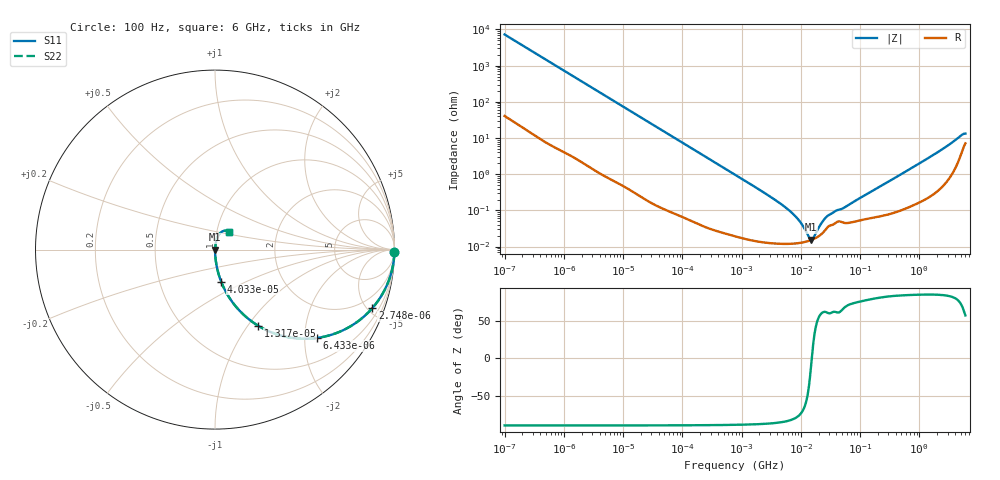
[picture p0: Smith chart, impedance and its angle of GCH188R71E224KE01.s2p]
!Murata Part Number: GCH188R71E224KE01
!These Parameters are Measured in Series Mode Connection
!Data Generated on Jun 19, 2026
!  o--ll--o
!Port1  Port2
!  o------o
!Operation Temp=25[degC], DC Bias Voltage=0[V]
!Freq. Start=100[Hz] Stop=6[GHz] 401[Steps]
# Hz S RI R 50
!Freq.(Hz) S11(Real) S11(Imag) S21(Real) S21(Imag) S12(Real) S12(Imag) S22(Real) S22(Imag)
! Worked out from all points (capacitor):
!   401 points, 100 Hz to 6 GHz, reference 50 ohm
!   read as one part in series: C = 218 nF near 109 Hz
!   lowest |Z| = 15.4 mohm at 14.88 MHz (marker M1)
!   series resonance near 15.31 MHz, so ESL is about 490 pH
!   S11 on the Smith chart (normalised r, x): 100 Hz: open; 2.748 kHz: 1.03, -5.36; 6.433 kHz: 1.01, -2.29; 13.17 kHz: 1.01, -1.12; 40.34 kHz: 1.00, -0.37; 6 GHz: 1.14, +0.22
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100  0.9997 -0.0137  0.000266 0.0137  0.000266 0.0137  0.9997 -0.0137
600  0.9929 -0.0813  0.00708 0.0813  0.00708 0.0813  0.9929 -0.0813
2008  0.9293 -0.2535  0.0707 0.2535  0.0707 0.2535  0.9293 -0.2535
2748  0.8762 -0.3265  0.1238 0.3265  0.1238 0.3265  0.8762 -0.3265
6433  0.5678 -0.4924  0.4322 0.4924  0.4322 0.4924  0.5678 -0.4924
13169  0.2415 -0.4248  0.7585 0.4248  0.7585 0.4248  0.2415 -0.4248
21550  0.1075 -0.3065  0.8925 0.3065  0.8925 0.3065  0.1075 -0.3065
40335  0.034 -0.1778  0.966 0.1778  0.966 0.1778  0.034 -0.1778
129199  0.00387 -0.0576  0.9961 0.0576  0.9961 0.0576  0.00387 -0.0576
774597  0.000287 -0.00971  0.9997 0.00971  0.9997 0.00971  0.000287 -0.00971
2967816  0.000131 -0.00246  0.9999 0.00246  0.9999 0.00246  0.000131 -0.00246
6075234  0.00012 -0.00106  0.9999 0.00106  0.9999 0.00106  0.00012 -0.00106
9506416  0.000126 -0.000493  0.9999 0.000493  0.9999 0.000493  0.000126 -0.000493
1.360128e7  0.000144 -0.000118  0.9999 0.000118  0.9999 0.000118  0.000144 -0.000118
1.487547e7  0.000151 -2.86e-05  0.9998 2.86e-05  0.9998 2.86e-05  0.000151 -2.86e-05
1.555665e7  0.000156 1.61e-05  0.9998 -1.61e-05  0.9998 -1.61e-05  0.000156 1.61e-05
2.327686e7  0.000236 0.000432  0.9998 -0.000432  0.9998 -0.000432  0.000236 0.000432
2.911731e7  0.000358 0.000634  0.9996 -0.000634  0.9996 -0.000634  0.000358 0.000634
3.124326e8  0.000826 0.00637  0.9992 -0.00637  0.9992 -0.00637  0.000826 0.00637
3.065283e9  0.0107 0.0613  0.9893 -0.0613  0.9893 -0.0613  0.0107 0.0613
5.016141e9  0.0437 0.1025  0.9563 -0.1025  0.9563 -0.1025  0.0437 0.1025
6e9  0.0765 0.0962  0.9235 -0.0962  0.9235 -0.0962  0.0765 0.0962
